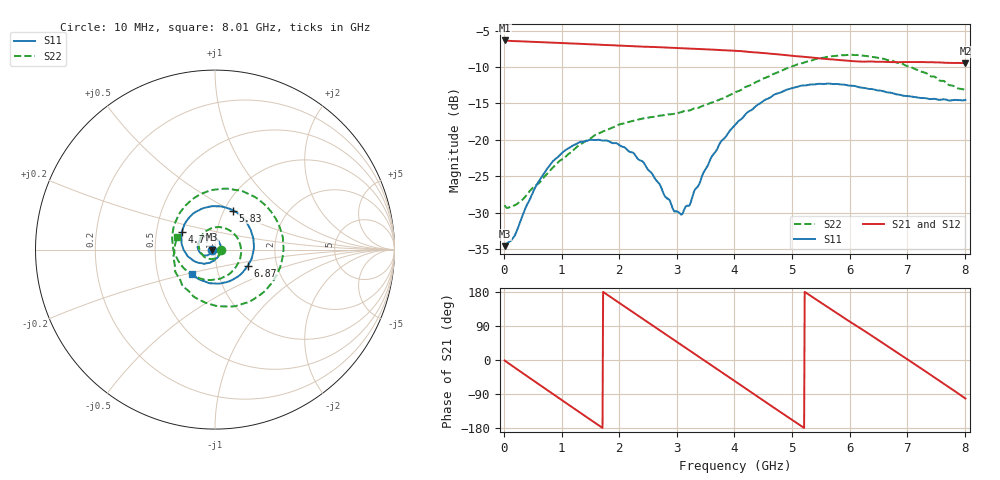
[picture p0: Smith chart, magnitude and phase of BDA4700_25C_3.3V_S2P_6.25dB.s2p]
!Agilent Technologies,E5071B,MY42404982,A.09.10
!Date: Mon Oct 20 18:05:37 2025
!Data & Calibration Information:
!Freq	S11:SOLT2(ON)	S21:SOLT2(ON)	S12:SOLT2(ON)	S22:SOLT2(ON)
# Hz S RI R 50
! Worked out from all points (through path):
!   801 points, 10 MHz to 8.01 GHz, reference 50 ohm
!   highest |S21| = -6.36 dB at 10 MHz (marker M1); lowest = -9.5 dB at 8.01 GHz (marker M2)
!   group delay of S21, straight-line fit = 284 ps
!   lowest |S11| = -34.6 dB at 10 MHz (marker M3), VSWR 1.04, Z = 48.2 - j0.0967 ohm
!   |S11| at or under -10 dB: start of sweep to end of sweep
!   |S22| runs from -29.4 to -8.3 dB; largest |S21 - S12| = 0.0056
!   S11 on the Smith chart (normalised r, x): 10 MHz: 0.96, -0.00; 4.77 GHz: 0.68, +0.14; 5.83 GHz: 1.10, +0.51; 6.87 GHz: 1.41, -0.27; 8.01 GHz: 0.75, -0.21
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1e7  -0.0186 -0.001  0.4807 -0.0105  0.4806 -0.0108  0.0355 -0.00276
3.3e8  -0.0239 -0.0194  0.3867 -0.2733  0.3861 -0.2733  0.0231 -0.0315
7.2e8  -0.0513 -0.0329  0.1108 -0.4534  0.111 -0.4532  -0.0209 -0.0529
1.02e9  -0.0792 -0.0221  -0.139 -0.4397  -0.1393 -0.4399  -0.0653 -0.0346
1.35e9  -0.0966 0.00954  -0.3584 -0.281  -0.3585 -0.2809  -0.0903 0.026
1.64e9  -0.0898 0.0443  -0.4457 -0.0624  -0.446 -0.0626  -0.0672 0.0875
1.93e9  -0.0638 0.0702  -0.4121 0.1668  -0.4121 0.1668  -0.000903 0.1234
2.32e9  -0.0158 0.0724  -0.2042 0.3871  -0.2043 0.3871  0.1013 0.0928
2.68e9  0.0216 0.0458  0.0691 0.4268  0.0685 0.4265  0.1455 -0.00753
2.95e9  0.031 0.00973  0.257 0.3422  0.2564 0.3414  0.1208 -0.0899
3.09e9  0.0291 -0.0102  0.3333 0.2649  0.3308 0.2668  0.0912 -0.1259
3.53e9  -0.0126 -0.0646  0.4151 -0.0475  0.4153 -0.0484  -0.0506 -0.1677
4.01e9  -0.106 -0.0686  0.2275 -0.339  0.2282 -0.3383  -0.1979 -0.0744
4.38e9  -0.1712 -0.00763  -0.0294 -0.3967  -0.0295 -0.3971  -0.2387 0.0724
4.77e9  -0.1839 0.0989  -0.2703 -0.2754  -0.2687 -0.2765  -0.1705 0.2376
5.35e9  -0.0621 0.2316  -0.3567 0.0854  -0.3569 0.0833  0.1103 0.3334
5.83e9  0.101 0.2178  -0.1695 0.3098  -0.1679 0.3096  0.3349 0.1787
6.24e9  0.197 0.1136  0.0684 0.3374  0.0736 0.336  0.372 -0.0624
6.68e9  0.2079 -0.0346  0.2821 0.1933  0.2829 0.1923  0.2252 -0.27
6.87e9  0.1815 -0.0922  0.329 0.0914  0.3291 0.0887  0.123 -0.3125
7.47e9  0.0219 -0.1898  0.2376 -0.2436  0.237 -0.2442  -0.1779 -0.2048
8.01e9  -0.1298 -0.1355  -0.0678 -0.3286  -0.0669 -0.3289  -0.2095 0.0694
